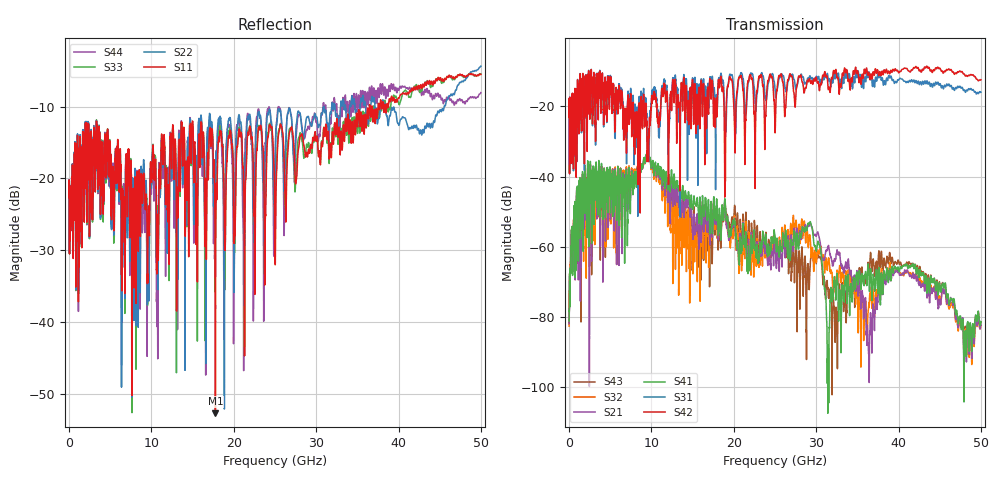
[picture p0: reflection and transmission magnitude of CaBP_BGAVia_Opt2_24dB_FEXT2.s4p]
!* Samtec Inc. NovaRay Examax Flyover System  *
!*  REV DATE  = 08/08/18  *
!*  TYPE  = TOUCHSTONE  *
!*  PORTS  = 4 port  *
!*  UNITS  = GHz  *
!*  DATA RANGE = DC  to 50 GHz; 10 MHz Step  *
!*  PARAMETER  = S  *
!*  FORMAT  = Real-Imaginary  *
!*  REFERENCE  = 50 ohms  *
!*  SOURCE  = HFSS  *
!*  VALIDATED  = No  *
!*  MANUFACTURER = SAMTEC  *
!*  INTERCONNECT = NVAx to EBCx to EBCx to NVAx  *
!*  [Full Channel NVAx to EBCx to EBCx to NVAx  with PCB Trace and BGA Via]  *
!*  BOUNDARY A  = Silicon BGA Ball Pad  *
!*  BOUNDARY B  = Silicon BGA Ball Pad  *
!*  NVAx (end a) ->>- (end b) NVAx  *
!*  Port 01 ->>- Port 02  *
!*  Port 03 ->>- Port 04  *
!***************************** CHANNEL MODEL ******************************************
# GHz S RI R 50
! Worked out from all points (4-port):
!   5000 points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, 10 MHz to 50 GHz, reference 50 ohm
!   strongest paths, dB at 10 MHz, 12.51 GHz, 25.01 GHz, 37.51 GHz, 50 GHz:
!     S42: -23.2, -15.1, -27.3, -10.1, -12.5
!     S31: -23.2, -14.5, -15.2, -10.7, -16.0
!     S41: -81.1, -41.3, -56.8, -72.5, -81.3
!     S21: -81.9, -44.8, -60.7, -73.9, -82.2
!     S32: -82.5, -50.4, -58.3, -70.8, -82.4
!     S43: -81.5, -45.1, -58.8, -65.8, -81.3
!   lowest |S11| = -52.7 dB at 17.77 GHz (marker M1), VSWR 1.00, Z = 49.8 - j0.145 ohm
!   |S11| at or under -10 dB: start of sweep to 36.46 GHz; 36.55 GHz to 36.75 GHz (204 MHz wide, 0.557 % of centre); 36.79 GHz to 37.51 GHz (722.9 MHz wide, 1.95 % of centre)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
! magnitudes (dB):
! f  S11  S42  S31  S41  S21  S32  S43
! 10 MHz  -22.7  -23.2  -23.2  -81.1  -81.9  -82.5  -81.5
! 780 MHz  -17.3  -18.6  -18.6  -53.2  -52.9  -51.7  -51.9
! 3.1 GHz  -13.9  -12.2  -12.3  -42.0  -45.1  -49.9  -45.3
! 17.77 GHz  -52.7  -25.4  -28.1  -51.5  -52.6  -53.1  -54.8
! 29.25 GHz  -16.3  -12.5  -11.3  -53.0  -53.5  -56.9  -66.3
! 31.44 GHz  -13.6  -14.4  -11.6  -91.4  -60.1  -64.8  -72.0
! 50 GHz  -5.5  -12.5  -16.0  -81.3  -82.2  -82.4  -81.3
